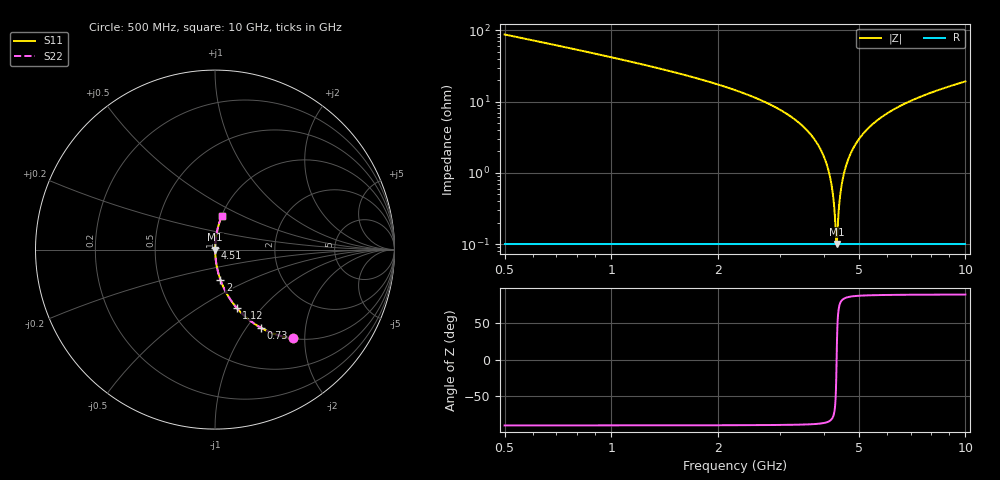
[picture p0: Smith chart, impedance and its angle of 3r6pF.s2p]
! Created Fri Jan 10 15:53:50 2014
# hz S db R 50
! 2 Port Network Data from SP1.SP block
! freq  dbS11  angS11  dbS21  angS21  dbS12  angS12  dbS22  angS22
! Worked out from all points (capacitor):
!   951 points, 500 MHz to 10 GHz, reference 50 ohm
!   read as one part in series: C = 3.6 pF near 540 MHz
!   lowest |Z| = 101 mohm at 4.33 GHz (marker M1)
!   series resonance near 4.329 GHz, so ESL is about 380 pH
!   S11 on the Smith chart (normalised r, x): 500 MHz: 1.00, -1.74; 730 MHz: 1.00, -1.18; 1.12 GHz: 1.00, -0.74; 2 GHz: 1.00, -0.35; 4.51 GHz: 1.00, +0.02; 10 GHz: 1.00, +0.38
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5e8  -3.65 -48.9  -2.46 41.1  -2.46 41.1  -3.65 -48.9
7.3e8  -5.90 -59.5  -1.30 30.4  -1.30 30.4  -5.90 -59.5
1.12e9  -9.24 -69.6  -0.56 20.2  -0.56 20.2  -9.24 -69.6
2e9  -15.33 -79.8  -0.14 9.9  -0.14 9.9  -15.33 -79.8
2.09e9  -15.92 -80.4  -0.12 9.2  -0.12 9.2  -15.92 -80.4
3.08e9  -23.02 -85.1  -0.03 4.0  -0.03 4.0  -23.02 -85.1
3.67e9  -29.41 -86.4  -0.01 1.9  -0.01 1.9  -29.41 -86.4
3.93e9  -34.08 -85.9  -0.01 1.1  -0.01 1.1  -34.08 -85.9
4.11e9  -39.47 -83.9  -0.01 0.6  -0.01 0.6  -39.47 -83.9
4.21e9  -44.78 -79.6  -0.01 0.3  -0.01 0.3  -44.78 -79.6
4.3e9  -55.42 -53.4  -0.01 0.1  -0.01 0.1  -55.42 -53.4
4.33e9  -59.91 3.3  -0.01 -0.0  -0.01 -0.0  -59.91 3.3
4.36e9  -54.99 55.4  -0.01 -0.1  -0.01 -0.1  -54.99 55.4
4.43e9  -46.33 77.7  -0.01 -0.3  -0.01 -0.3  -46.33 77.7
4.51e9  -41.48 82.6  -0.01 -0.5  -0.01 -0.5  -41.48 82.6
4.62e9  -37.50 84.9  -0.01 -0.8  -0.01 -0.8  -37.50 84.9
4.78e9  -33.86 86.0  -0.01 -1.2  -0.01 -1.2  -33.86 86.0
5.25e9  -28.05 86.3  -0.02 -2.3  -0.02 -2.3  -28.05 86.3
5.91e9  -23.82 85.4  -0.03 -3.7  -0.03 -3.7  -23.82 85.4
6.84e9  -20.34 83.9  -0.05 -5.5  -0.05 -5.5  -20.34 83.9
8.42e9  -16.80 81.3  -0.10 -8.3  -0.10 -8.3  -16.80 81.3
1e10  -14.51 78.9  -0.17 -10.8  -0.17 -10.8  -14.51 78.9
